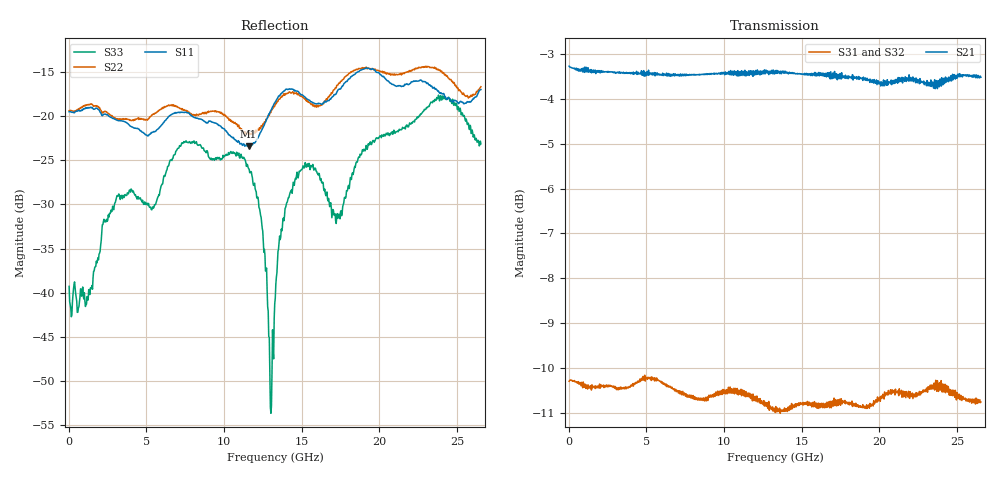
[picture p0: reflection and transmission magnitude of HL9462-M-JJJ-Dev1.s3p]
! 4/7/2020 11:13:34 AM
! H:\PRODUCTION_DATA\TEMP_S3P.S3P
! CHANNEL.1
! TR.MEASUREMENT
! CORRECTED.DATA
# GHZ S RI R 50.0
! FREQ.GHZ  S11RE  S11IM  S12RE  S12IM  S13RE  S13IM
!  S21RE  S21IM  S22RE  S22IM  S23RE  S23IM
!  S31RE  S31IM  S32RE  S32IM  S33RE  S33IM
!; PortSelection: Port_123
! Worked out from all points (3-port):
!   758 points, 35 MHz to 26.53 GHz, reference 50 ohm
!   strongest paths, dB at 35 MHz, 6.65 GHz, 13.3 GHz, 19.91 GHz, 26.53 GHz:
!     S21: -3.3, -3.5, -3.4, -3.6, -3.5
!     S31: -10.3, -10.4, -11.0, -10.7, -10.8
!     S32: -10.3, -10.5, -10.9, -10.8, -10.8
!   lowest |S11| = -23.4 dB at 11.59 GHz (marker M1), VSWR 1.14, Z = 46.8 - j5.72 ohm
!   |S11| at or under -10 dB: start of sweep to end of sweep
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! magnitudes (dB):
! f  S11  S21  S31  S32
! 35 MHz  -19.5  -3.3  -10.3  -10.3
! 7.385 GHz  -19.6  -3.5  -10.6  -10.7
! 11.59 GHz  -23.4  -3.4  -10.6  -10.8
! 12.43 GHz  -21.6  -3.5  -10.7  -10.8
! 12.98 GHz  -19.5  -3.4  -10.8  -10.9
! 13.3 GHz  -18.4  -3.4  -11.0  -10.9
! 15.15 GHz  -17.8  -3.5  -10.8  -11.0
! 17.29 GHz  -17.2  -3.6  -10.7  -10.8
! 23.73 GHz  -17.1  -3.8  -10.3  -10.7
! 26.53 GHz  -17.0  -3.5  -10.8  -10.8
